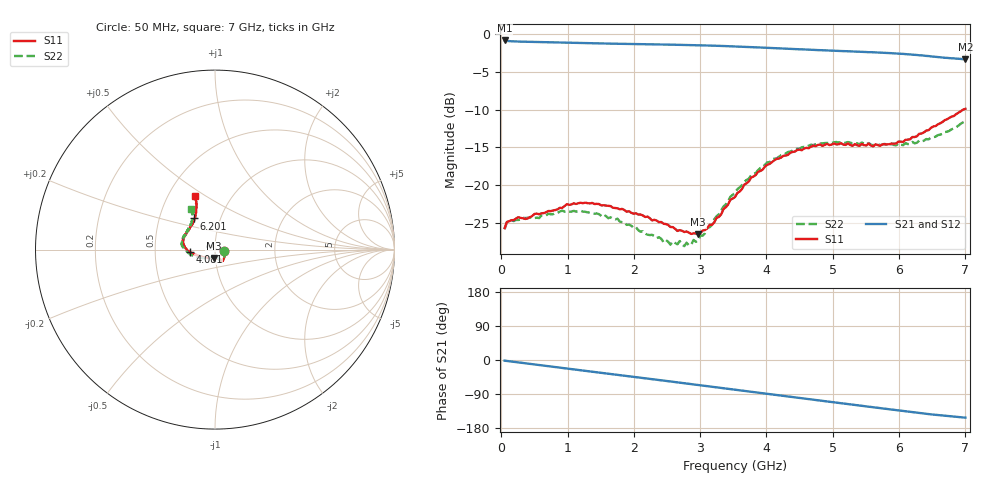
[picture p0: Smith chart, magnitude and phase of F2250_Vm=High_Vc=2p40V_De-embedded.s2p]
! Integrated Device Technology
! Corporate Headquarters
! 6024 Silver Creek Valley Road
! San Jose, CA 95138  USA
! Phone:  1-408-284-8200
! Toll Free:  1-800-223-1366
! Webpage:  http://www.idt.com/
! Timing and RF Division
! 515 Groton Road, Suite 102
! Westford, MA 01886-6024
! Device:  F2250
! Description: Voltage Variable RF Attenuator
! Frequency:  50.0 -  6000.00 MHz
! Package:  3x3 mm Thin QFN Plastic Package: 16 pin
! Ports:  2 RF, 3 DC
!  Pin  1  = GND
!  Pin  2  = NC
!  Pin  3  = RF1  = Port 1
!  Pin  4  = NC
!  Pin  5  = GND
!  Pin  6  = GND
!  Pin  7  = GND
!  Pin  8  = GND
!  Pin  9  = NC
!  Pin 10  = RF2  = Port 2
!  Pin 11  = NC
!  Pin 12  = GND
!  Pin 13  = GND
!  Pin 14  = VCNTRL
!  Pin 15  = VDD
!  Pin 16  = VMODE
! Vcntrl:  2.400 Volts
! Vmode:  +3.300 Volts
! Vdd:  +3.30  Volts
! Current:  1.314 mA
! Data:  The device was measured on a the F2250 evaluation board which has
!  individual transmission lines to the RF pins.  Data was collected
!  using a calibrated network analyzer.  The evaluation board was
!  de-embedded using a TRL calibration technique.
!  The reference plane is the edge of the package pin.
! Misc:  SN 10
!  Action Tracker AT0258
! Date Measured:  2014-11-26
! Date:  2015-10-15  MJV
! Note:
!  Integrated Device Technology supplies this data as a sample of measured
!  data at the package pin for this product.  Your particular data for this
!  product may vary.
!  Data was taken at 25 degrees C.
!  Integrated Device Technology reserves the right to change this data at anytime.
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# GHz S dB R 50
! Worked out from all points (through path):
!   201 points, 50 MHz to 7 GHz, reference 50 ohm
!   highest |S21| = -0.89 dB at 50 MHz (marker M1); lowest = -3.4 dB at 7 GHz (marker M2)
!   group delay of S21, straight-line fit = 61.2 ps
!   lowest |S11| = -26.5 dB at 2.969 GHz (marker M3), VSWR 1.10, Z = 49.2 - j4.63 ohm
!   |S11| at or under -10 dB: start of sweep to 6.969 GHz
!   |S22| runs from -28.0 to -11.6 dB; largest |S21 - S12| = 0.002
!   S11 on the Smith chart (normalised r, x): 50 MHz: 1.11, -0.02; 4.081 GHz: 0.75, -0.02; 6.201 GHz: 0.75, +0.27; 7 GHz: 0.68, +0.45
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0.05  -25.63 -10.6  -0.89 -1.8  -0.89 -1.8  -25.79 -10.8
0.1195  -24.73 -10.3  -0.99 -3.2  -0.99 -3.2  -24.67 -8.9
0.57125  -23.81 -31.3  -1.10 -13.3  -1.10 -13.3  -24.31 -31.4
0.91875  -22.98 -50.1  -1.17 -21.0  -1.17 -21.1  -23.33 -51.0
1.2315  -22.35 -57.8  -1.24 -27.9  -1.24 -27.9  -23.46 -61.5
1.75275  -23.03 -64.8  -1.33 -39.1  -1.33 -39.1  -24.40 -67.8
2.37825  -24.85 -64.5  -1.42 -52.8  -1.42 -52.8  -26.84 -66.8
2.552  -25.49 -69.3  -1.45 -56.7  -1.45 -56.7  -27.82 -73.2
2.691  -25.91 -77.4  -1.47 -59.8  -1.47 -59.8  -27.34 -81.0
2.7605  -26.15 -79.6  -1.49 -61.3  -1.49 -61.3  -28.02 -85.5
2.969  -26.48 -97.6  -1.53 -66.0  -1.53 -66.0  -27.25 -105.0
3.1775  -25.20 -120.7  -1.57 -70.7  -1.57 -70.7  -25.23 -126.8
3.525  -21.54 -152.7  -1.68 -78.5  -1.68 -78.6  -20.96 -148.8
3.76825  -18.97 -164.7  -1.77 -84.0  -1.77 -84.1  -18.69 -159.7
4.081  -16.95 -175.7  -1.90 -91.0  -1.90 -91.0  -16.72 -171.5
4.4285  -15.54 176.0  -2.03 -98.6  -2.04 -98.7  -15.20 178.6
4.7065  -14.77 169.1  -2.13 -104.8  -2.13 -104.8  -14.69 172.9
5.054  -14.61 160.9  -2.26 -112.5  -2.26 -112.5  -14.28 165.9
5.85325  -14.57 135.1  -2.56 -130.0  -2.56 -130.1  -14.69 147.2
6.20075  -13.62 123.6  -2.77 -137.7  -2.77 -137.8  -14.27 138.2
6.54825  -12.19 115.6  -3.04 -144.7  -3.04 -144.9  -13.60 126.9
7  -9.91 110.8  -3.37 -152.1  -3.38 -152.2  -11.56 120.6
